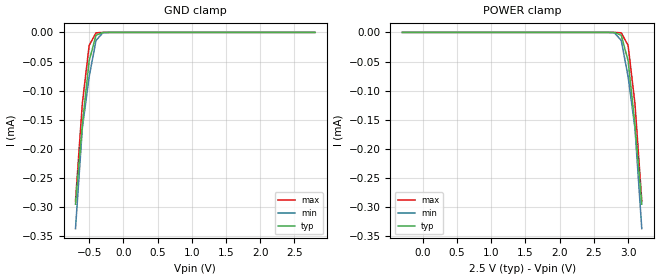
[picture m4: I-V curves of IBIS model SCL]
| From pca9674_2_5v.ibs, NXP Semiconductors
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[Model]   SCL
Model_type Input
Vinh=1.5
Vinl=0.75
C_comp   5p   4.8p   5.2p
[Model Spec]
Vinh   2.31   1.61   3.85
Vinl   0.99   0.69   1.65
[Temperature Range] 27   85   -40
[Voltage Range]   2.5   2.2   2.8
[GND Clamp]
-700mV    -295uA     -337uA     -289.5uA
-600mV    -158.8uA   -164.3uA   -122uA
-500mV    -48.62uA   -75.94uA   -22.35uA
-400mV    -4.926uA   -13.83uA   -710.6nA
-300mV    -138.4nA   -722.3nA   -7.551nA
2.8V      6.71pA     20.63pA    5.609pA
[POWER Clamp]
-300mV    6.71pA     20.63pA    5.609pA
2.8V      -138.4nA   -722.3nA   -7.551nA
2.9V      -4.926uA   -13.83uA   -710.6nA
3V        -48.62uA   -75.94uA   -22.35uA
3.1V      -158.8uA   -164.3uA   -122uA
3.2V      -295uA     -337uA     -289.5uA
